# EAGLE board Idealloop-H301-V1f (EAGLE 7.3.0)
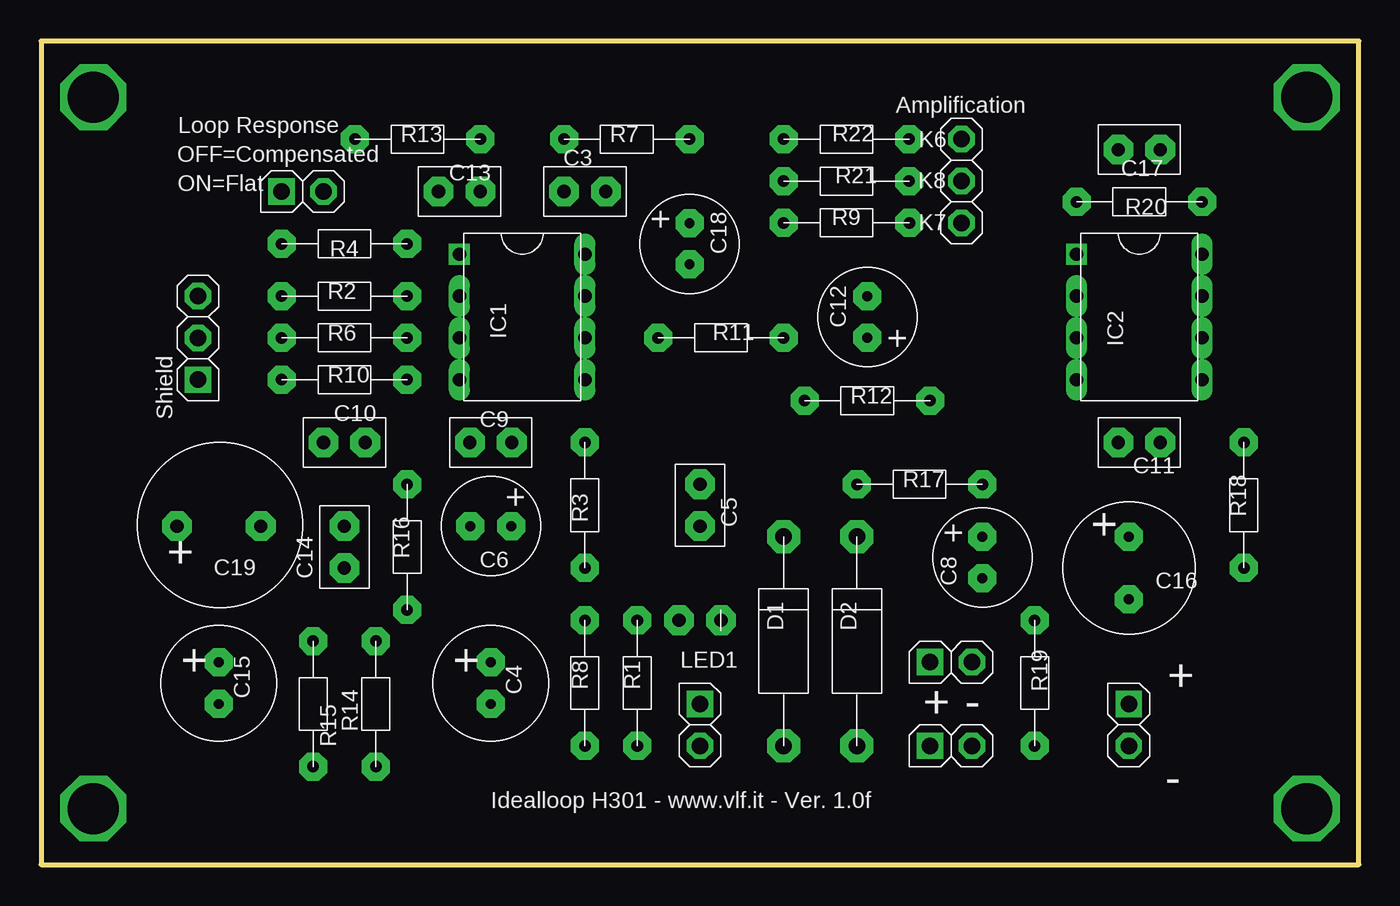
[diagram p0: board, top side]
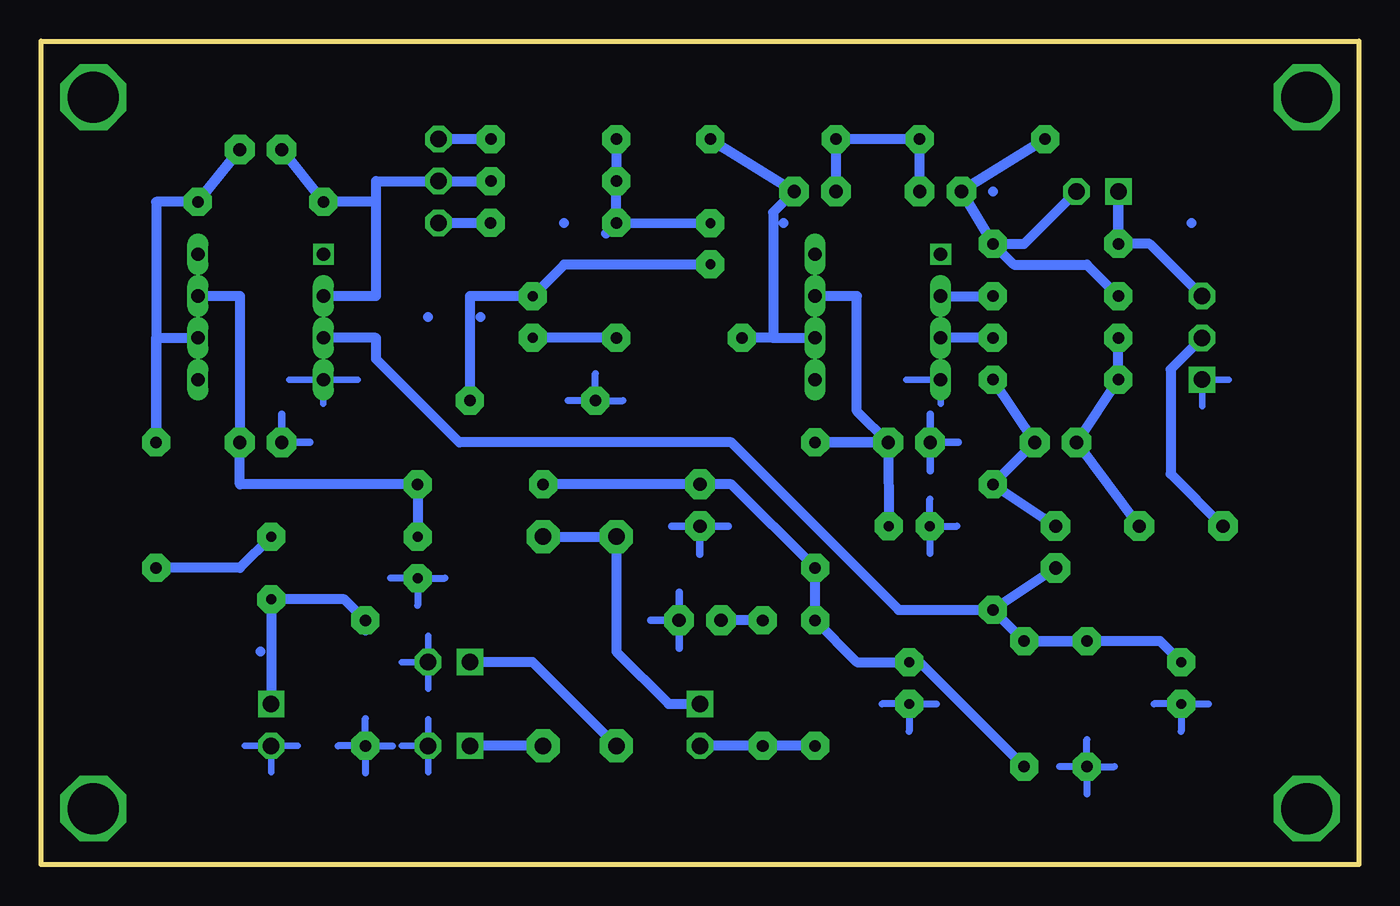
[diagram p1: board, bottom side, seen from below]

Size 80 x 50 mm. Coordinates in mm from the lower left corner, seen from the top.
Outline: 0,50 0,0 80,0 80,50 0,50
Copper layers 16: Bottom 0.035mm
Design rules "TARGET3001!": minimum track width 0.4mm, minimum drill 0.6mm, track to track 0.5mm, track to pad 0.5mm, pad to pad 0.5mm, via to via 0.5mm, smd to smd 0mm, copper to edge 0mm, drill to drill 0.3mm, minimum pad ring 0.235mm, minimum via ring 0.45mm, stop-mask expansion 4mil, vias tented up to drill 0mil, thermal gap 10mil

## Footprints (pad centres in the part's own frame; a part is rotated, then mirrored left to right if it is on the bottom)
3X5R2,54_46 = drill 0.8 pad 1.8 octagon: 1 1.27,0; 2 -1.27,0
D7R2,54_ELKO_23 = drill 0.6 pad 1.7 octagon: 1 0,1.27; 2 0,-1.27
3X5R2,54_43 = drill 0.8 pad 1.8 octagon: 1 0,-1.27; 2 0,1.27
D6R2,54_ELKO_61 = drill 0.6 pad 1.7 octagon: 1 1.25,0; 2 -1.25,0
D6R2,54_ELKO_62 = drill 0.6 pad 1.7 octagon: 1 0,1.25; 2 0,-1.25
3X5R2,54_47 = drill 0.8 pad 1.8 octagon: 1 1.27,0; 2 -1.27,0
3X5R2,54_48 = drill 0.8 pad 1.8 octagon: 1 -1.27,0; 2 1.27,0
3X5R2,54_44 = drill 0.8 pad 1.8 octagon: 1 -1.27,0; 2 1.27,0
D6R2,54_ELKO_24 = drill 0.6 pad 1.7 octagon: 1 0,-1.25; 2 0,1.25
3X5R2,54_41 = drill 0.8 pad 1.8 octagon: 1 -1.27,0; 2 1.27,0
3X5R2,54_42 = drill 0.8 pad 1.8 octagon: 1 0,-1.27; 2 0,1.27
D7R2,54_ELKO_27 = drill 0.6 pad 1.7 octagon: 1 0,1.27; 2 0,-1.27
D8R3,81_ELKO_26 = drill 0.6 pad 1.7 octagon: 1 0,1.905; 2 0,-1.905
3X5R2,54_45 = drill 0.8 pad 1.8 octagon: 1 1.27,0; 2 -1.27,0
D6R2,54_ELKO_25 = drill 0.6 pad 1.7 octagon: 1 0,1.25; 2 0,-1.25
D10R5,08_ELKO_22 = drill 0.8 pad 1.8 octagon: 1 -2.54,0; 2 2.54,0
D_RM12,7_DM3_30 = drill 1 pad 2 octagon: 1 0,-6.35; 2 0,6.35
D_RM12,7_DM3_29 = drill 1 pad 2 octagon: 1 0,-6.35; 2 0,6.35
DIL8_0 = drill 0.8 pad 1.27 square: 1 -3.81,3.81 | drill 0.8 pad 1.27 long: 2 -3.81,1.27; 3 -3.81,-1.27; 4 -3.81,-3.81; 5 3.81,-3.81; 6 3.81,-1.27; 7 3.81,1.27; 8 3.81,3.81
DIL8_40 = drill 0.8 pad 1.27 square: 1 -3.81,3.81 | drill 0.8 pad 1.27 long: 2 -3.81,1.27; 3 -3.81,-1.27; 4 -3.81,-3.81; 5 3.81,-3.81; 6 3.81,-1.27; 7 3.81,1.27; 8 3.81,3.81
Stiftleiste_1x02_G_2,54_51 = drill 1 pad 1.6 square: 1 0,0 | drill 1 pad 1.6 octagon: 2 2.54,0
Stiftleiste_1x03_G_2,54_37 = drill 1 pad 1.6 square: 1 0,0 | drill 1 pad 1.6 octagon: 2 0,2.54; 3 0,5.08
Stiftleiste_1x02_G_2,54_52 = drill 1 pad 1.6 square: 1 0,0 | drill 1 pad 1.6 octagon: 2 0,-2.54
Stiftleiste_1x02_G_2,54_53 = drill 1 pad 1.6 square: 1 0,0 | drill 1 pad 1.6 octagon: 2 2.54,0
Stiftleiste_1x02_G_2,54_39 = drill 1 pad 1.6 square: 1 0,0 | drill 1 pad 1.6 octagon: 2 0,-2.54
Stiftleiste_1x01_G_2,54_54 = drill 1 pad 1.6 octagon: 1 0,0
Stiftleiste_1x01_G_2,54_55 = drill 1 pad 1.6 octagon: 1 0,0
Stiftleiste_1x01_G_2,54_56 = drill 1 pad 1.6 octagon: 1 0,0
Stiftleiste_1x02_G_2,54_57 = drill 1 pad 1.6 square: 1 0,0 | drill 1 pad 1.6 octagon: 2 2.54,0
LED_3MM_ROT_28 = drill 0.8 pad 1.8 octagon: 1 -1.27,0; 2 1.27,0
0204_MET_11 = drill 0.7 pad 1.7 octagon: 1 0,-3.81; 2 0,3.81
0204_MET_2 = drill 0.7 pad 1.7 octagon: 1 -3.81,0; 2 3.81,0
0204_MET_20 = drill 0.7 pad 1.7 octagon: 1 0,-3.81; 2 0,3.81
0204_MET_1 = drill 0.7 pad 1.7 octagon: 1 -3.81,0; 2 3.81,0
0204_MET_3 = drill 0.7 pad 1.7 octagon: 1 -3.81,0; 2 3.81,0
0204_MET_5 = drill 0.7 pad 1.7 octagon: 1 -3.81,0; 2 3.81,0
0204_MET_10 = drill 0.7 pad 1.7 octagon: 1 0,-3.81; 2 0,3.81
0204_MET_15 = drill 0.7 pad 1.7 octagon: 1 3.825,0; 2 -3.81,0
0204_MET_6 = drill 0.7 pad 1.7 octagon: 1 -3.81,0; 2 3.81,0
0204_MET_12 = drill 0.7 pad 1.7 octagon: 1 3.81,0; 2 -3.81,0
0204_MET_21 = drill 0.7 pad 1.7 octagon: 1 -3.81,0; 2 3.81,0
0204_MET_4 = drill 0.7 pad 1.7 octagon: 1 -3.81,0; 2 3.81,0
0204_MET_9 = drill 0.7 pad 1.7 octagon: 1 0,-3.81; 2 0,3.81
0204_MET_8 = drill 0.7 pad 1.7 octagon: 1 0,3.81; 2 0,-3.81
0204_MET_7 = drill 0.7 pad 1.7 octagon: 1 0,3.81; 2 0,-3.81
0204_MET_19 = drill 0.7 pad 1.7 octagon: 1 -3.81,0; 2 3.81,0
0204_MET_17 = drill 0.7 pad 1.7 octagon: 1 0,-3.81; 2 0,3.81
0204_MET_18 = drill 0.7 pad 1.7 octagon: 1 0,-3.81; 2 0,3.81
0204_MET_16 = drill 0.7 pad 1.7 octagon: 1 3.81,0; 2 -3.81,0
0204_MET_13 = drill 0.7 pad 1.7 octagon: 1 3.81,0; 2 -3.81,0
0204_MET_14 = drill 0.7 pad 1.7 octagon: 1 3.81,0; 2 -3.81,0

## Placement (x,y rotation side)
C3  220pF  [3X5R2,54_46]  33.02,40.88 0 top
C4  100µF  [D7R2,54_ELKO_23]  27.3,11.03 0 top
C5  100nF  [3X5R2,54_43]  40,21.82 0 top
C6  1µF  [D6R2,54_ELKO_61]  27.3,20.55 0 top
C8  1µF  [D6R2,54_ELKO_62]  57.14,18.65 0 top
C9  100nF  [3X5R2,54_47]  27.3,25.64 0 top
C10  220pF  [3X5R2,54_48]  18.41,25.64 0 top
C11  100nF  [3X5R2,54_44]  66.67,25.64 0 top
C12  4.7µF  [D6R2,54_ELKO_24]  50.16,33.26 0 top
C13  47nF  [3X5R2,54_41]  25.39,40.88 0 top
C14  47nF  [3X5R2,54_42]  18.41,19.29 0 top
C15  100µF  [D7R2,54_ELKO_27]  10.79,11.03 0 top
C16  220µF  [D8R3,81_ELKO_26]  66.03,18.02 0 top
C17  100pF  [3X5R2,54_45]  66.67,43.41 0 top
C18  4.7µF  [D6R2,54_ELKO_25]  39.37,37.7 0 top
C19  470µF  [D10R5,08_ELKO_22]  10.79,20.55 0 top
D1  1N4001  [D_RM12,7_DM3_30]  45.08,13.57 0 top
D2  1N4001  [D_RM12,7_DM3_29]  49.52,13.57 0 top
DRILL1  Bohrung  [Bohrung_58]  76.83,46.59 0 top
DRILL2  Bohrung  [Bohrung_59]  76.83,3.41 0 top
DRILL3  Bohrung  [Bohrung_65]  3.17,46.59 0 top
DRILL4  Bohrung  [Bohrung_60]  3.17,3.41 0 top
IC1  AD797  [DIL8_0]  29.2,33.26 0 top
IC2  OP27GPZ  [DIL8_40]  66.67,33.26 0 top
K1  9-24 V-DC  [Stiftleiste_1x02_G_2,54_51]  53.97,7.22 0 top
K2  Loop IN  [Stiftleiste_1x03_G_2,54_37]  9.52,29.45 0 top
K3  Output  [Stiftleiste_1x02_G_2,54_52]  66.03,9.76 0 top
K4  9 V Bat.  [Stiftleiste_1x02_G_2,54_53]  53.97,12.3 0 top
K5  ON/OFF  [Stiftleiste_1x02_G_2,54_39]  40,9.76 0 top
K6  Mid  [Stiftleiste_1x01_G_2,54_54]  55.88,44.05 0 top
K7  High  [Stiftleiste_1x01_G_2,54_55]  55.88,38.97 0 top
K8  Low  [Stiftleiste_1x01_G_2,54_56]  55.88,41.51 0 top
K9  Filter Flat/Comp.  [Stiftleiste_1x02_G_2,54_57]  14.6,40.88 0 top
LED1  LED_ROT_3MM  [LED_3MM_ROT_28]  40,14.84 0 top
R1  2.2K  [0204_MET_11]  36.19,11.03 0 top
R2  22  [0204_MET_2]  18.41,34.52 0 top
R3  3.3  [0204_MET_20]  33.02,21.82 0 top
R4  2.2K  [0204_MET_1]  18.41,37.7 0 top
R6  22  [0204_MET_3]  18.41,31.98 0 top
R7  27k  [0204_MET_5]  35.55,44.05 0 top
R8  10  [0204_MET_10]  33.02,11.03 0 top
R9  1.2k  [0204_MET_15]  48.89,38.97 0 top
R10  27k  [0204_MET_6]  18.41,29.45 0 top
R11  1K  [0204_MET_12]  41.27,31.98 0 top
R12  10k  [0204_MET_21]  50.16,28.18 0 top
R13  220k  [0204_MET_4]  22.86,44.05 0 top
R14  10k  [0204_MET_9]  20.32,9.76 0 top
R15  10k  [0204_MET_8]  16.5,9.76 0 top
R16  220k  [0204_MET_7]  22.22,19.29 0 top
R17  3.3  [0204_MET_19]  53.34,23.09 0 top
R18  1k  [0204_MET_17]  73.02,21.82 0 top
R19  10k  [0204_MET_18]  60.32,11.03 0 top
R20  100k  [0204_MET_16]  66.67,40.24 0 top
R21  220k  [0204_MET_13]  48.89,41.51 0 top
R22  22k  [0204_MET_14]  48.89,44.05 0 top

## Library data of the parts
C3-C6 C8-C19 D1 D2 DRILL1-DRILL4 IC1 IC2 K1-K9 LED1 R1-R4 R6-R22 = TARGET3001!_V18.2.0.34

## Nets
A: D1.1 K4.1
GND: C4.2 C5.1 C6.2 C8.2 C9.2 C11.1 C15.2 K1.2 K2.1 K3.2 K4.2 LED1.2 R12.1 R15.2 R19.1
Loop1: K2.3 K9.1 R4.1
Loop2: C19.1 K2.2
Sig$1: IC1.2 R2.2
Sig$2: IC1.3 R6.2
Sig$3: C10.2 C14.2 R10.2 R16.1
Sig$4: C10.1 C19.2 R6.1 R10.1
Sig$5: LED1.1 R1.2
Sig$6: C12.1 R11.1
Sig$7: C12.2 C18.2 R12.2
Sig$8: C18.1 R9.2 R21.2 R22.2
Sig$9: C17.2 IC2.2 K8.1 R20.2 R21.1
Sig$10: C17.1 IC2.6 R18.2 R20.1
Sig$12: C3.2 C13.2 R7.1 R13.2
Sig$16: C13.1 K9.2 R2.1 R4.2 R13.1
Sig$17: D1.2 D2.2 K5.1
Sig$18: D2.1 K1.1
Sig$19: C6.1 C9.1 R3.2
Sig$20: K5.2 R1.1 R8.1
Sig$21: C8.1 C11.2 R17.2
Sig$22: C14.1 C15.1 IC2.3 R14.2 R15.1 R16.2
Sig$23: C4.1 C5.2 R3.1 R8.2 R14.1 R17.1
Sig$25: K6.1 R22.1
Sig$26: K7.1 R9.1
Sig$27: C3.1 IC1.6 R7.2 R11.2
Sig$28: C16.2 K3.1 R19.2
Sig$29: C16.1 R18.1
V+: IC1.7 IC2.7
V-: IC1.4 IC2.4

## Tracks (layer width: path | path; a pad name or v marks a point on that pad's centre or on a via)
A
  Bottom 0.6: D1.1 50.16,12.3 K4.1
GND
  Bottom 0.4: 27.48,29.45 25.39,29.45 25.39,28 | 7.91,29.45 K2.1 9.52,27.84 | 62.86,29.45 64.94,29.45 | 62.86,29.45 62.86,28 | K1.2 58.12,7.22 | K1.2 56.51,8.83 | K1.2 56.51,5.61 | K3.2 67.64,7.22 | K3.2 64.42,7.22 | K3.2 66.03,5.61 | K4.2 58.12,12.3 | K4.2 56.51,13.91 | K4.2 56.51,10.69 | 62.86,29.45 60.78,29.45
  Bottom 0.425: R15.2 18.16,5.95 | R15.2 16.5,7.61 | R15.2 14.84,5.95 | R15.2 16.5,4.29 | R19.1 61.98,7.22 | R19.1 60.32,8.88 | R19.1 58.66,7.22 | R19.1 60.32,5.56 | R12.1 48.01,28.18 | R12.1 46.35,29.84 | R12.1 44.69,28.18 | C4.2 28.96,9.76 | C4.2 27.3,8.1 | C15.2 12.45,9.76 | C15.2 9.13,9.76 | C15.2 10.79,8.1 | C6.2 26.05,22.21 | C6.2 24.39,20.55 | C6.2 26.05,18.89 | C8.2 58.8,17.4 | C8.2 55.48,17.4 | C8.2 57.14,15.74 | C4.2 25.64,9.76
  Bottom 0.45: LED1.2 42.98,14.84 | LED1.2 41.27,16.55 | LED1.2 41.27,13.13 | C5.1 41.71,20.55 | C5.1 38.29,20.55 | C5.1 40,18.84 | 65.4,27.34 C11.1 63.69,25.64 | C9.2 26.03,27.34 | C9.2 24.32,25.64 | C9.2 26.03,23.93
Loop1
  Bottom 0.6: R4.1 K9.1 R4.1 | R4.1 | K2.3 | K2.3 12.7,37.7 R4.1 | 10.16,38.97
Loop2
  Bottom 0.6: C19.1 11.43,23.73 11.43,30.08 K2.2
Sig$1
  Bottom 0.6: IC1.2 R2.2
Sig$2
  Bottom 0.6: R6.2 IC1.3
Sig$3
  Bottom 0.6: C14.2 | C10.2 R16.1 | R16.1 C10.2 | R10.2 C10.2 | R16.1 C14.2
Sig$4
  Bottom 0.6: R6.1 R10.1 C10.1 | C10.1 | C19.2 | C10.1 | C19.2 C10.1
Sig$5
  Bottom 0.6: R1.2 | R1.2 | R1.2 LED1.1
Sig$6
  Bottom 0.6: R11.1 C12.1
Sig$7
  Bottom 0.6: 39.37,36.43 48.26,36.43 C12.2 53.97,34.52 R12.2
Sig$8
  Bottom 0.6: R9.2 R21.2 | R9.2 R21.2 | R9.2 C18.1 | R22.2 R21.2 | 45.72,38.34 | 46.35,28.18
Sig$9
  Bottom 0.6: C17.2 R20.2 | R21.1 K8.1 59.69,41.51 59.69,40.24 | 59.69,40.24 59.69,34.52 IC2.2 | 59.69,40.24 R20.2 | 59.69,40.24 R20.2 | 53.34,33.26 | 56.51,33.26
Sig$10
  Bottom 0.6: R20.1 C17.1 R20.1 | R20.1 73.02,40.24 73.02,31.98 | 73.02,31.98 R18.2 73.02,31.98 | 73.02,31.98 IC2.6 | 73.02,27.54 | 73.02,27.54
Sig$11
  Bottom 0.6: 48.26,38.97
Sig$12
  Bottom 0.6: C13.2 R13.2 R7.1 C3.2 | 22.22,40.88
Sig$16
  Bottom 0.6: R13.1 | R2.1 | R13.1 | C13.1 R4.2 | C13.1 R4.2 | R4.2 20.32,37.7 K9.2 | R13.1 | R13.1 | C13.1 R4.2 | R2.1 16.5,36.43 20.95,36.43 R4.2 | R13.1 C13.1 | R13.1 C13.1 | R13.1 C13.1 | R13.1 C13.1 | 14.6,39.61
Sig$17
  Bottom 0.6: D2.2 D1.2 45.08,12.94 41.91,9.76 K5.1
Sig$18
  Bottom 0.6: D2.1 K1.1
Sig$19
  Bottom 0.6: C9.1 C6.1 | R3.2 C9.1 | R3.2 | 33.02,34.52 30.48,34.52 30.48,27.54 C9.1 | C9.1 R3.2
Sig$20
  Bottom 0.6: K5.2 R1.1 R8.1
Sig$21
  Bottom 0.6: R17.2 C8.1 R17.2 | 70.48,34.52 67.94,34.52 C11.2 67.94,23.09 R17.2 | R17.2 | R17.2 | R17.2
Sig$22
  Bottom 0.6: R16.2 R14.2 | R14.2 R15.1 R14.2 | R16.2 27.94,15.47 38.09,25.64 54.61,25.64 59.69,30.71 59.69,31.98 IC2.3 | C14.1 | C15.1 12.06,13.57 R14.2 | R16.2 C14.1
Sig$23
  Bottom 0.6: R8.2 30.48,12.3 C4.1 | R8.2 R3.1 | R17.1 C5.2 38.09,23.09 R3.1 | R14.1 26.66,12.3 C4.1 | R14.1 | R14.1 | C4.1 | R8.2 R3.1
Sig$25
  Bottom 0.6: R22.1 K6.1
Sig$26
  Bottom 0.6: K7.1 R9.1
Sig$27
  Bottom 0.6: 34.92,38.97 | 35.55,31.98 IC1.6 | 34.92,38.97 | 35.55,39.61 35.55,31.98 | 35.55,39.61 35.55,31.98 | 35.55,39.61 35.55,31.98 | 35.55,39.61 C3.1 | 35.55,39.61 C3.1 | 35.55,39.61 C3.1 | R7.2 C3.1 | R7.2 C3.1 | R7.2 C3.1 | 35.55,31.98 R11.2
Sig$28
  Bottom 0.6: C16.2 K3.1 | R19.2 | R19.2 | 61.59,16.11 C16.2 | 61.59,16.11 C16.2 | 61.59,16.11 R19.2 | 61.59,16.11 R19.2 | 60.32,14.21 | 66.67,12.94
Sig$29
  Bottom 0.6: C16.1 67.94,18.02 R18.1
WITHOUT_SIGNAL  (via drill 3.1 pad 4)
  other vias: 3.17,46.59 76.83,46.59 3.17,3.41 76.83,3.41

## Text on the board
tPlace: Amplification | Loop Response | OFF=Compensated | ON=Flat | Shield | + | + | - | - | Idealloop H301 - www.vlf.it - Ver. 1.0f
